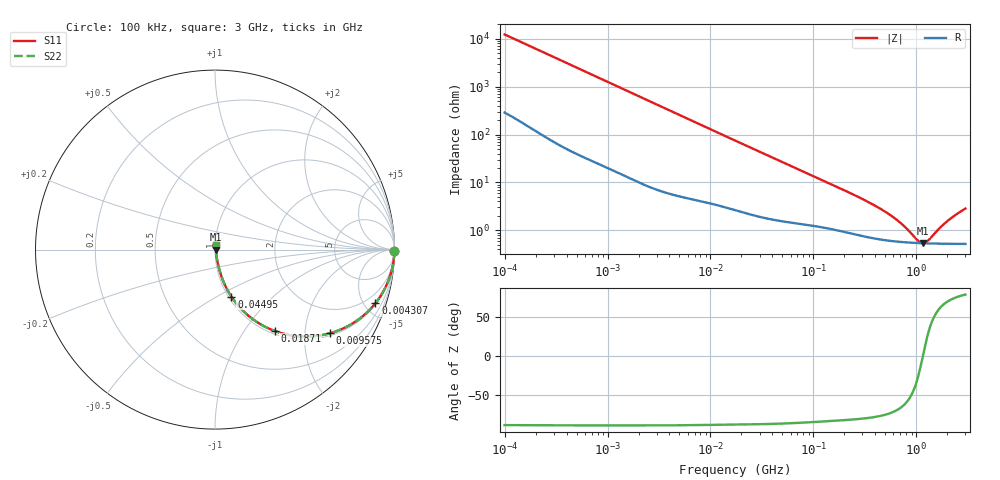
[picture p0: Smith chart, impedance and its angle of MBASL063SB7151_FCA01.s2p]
! MBASL063SB7151_FCA01  S-PARAMETER MODEL  ( Standard Model )
! Model Generated by TAIYO YUDEN Corporation (http://www.ty-top.com)
! Version 3.0
! TAIYO YUDEN Control No. 231201
! Copyright(c) 2020 TAIYO YUDEN CO.,LTD. All Rights Reserved.
! Product Description (link to TY-COMPAS)
! https://ds.yuden.co.jp/TYCOMPAS/or/detail?pn=MBASL063SB7151KFCA01&u=M
! Products Name : Multilayer Ceramic Capacitors
! Characteristics :
!  Capacitance : 150 [pF] , Rated Voltage : 10 [V] , TCC : X7R
!  Case Size : 0.6 x 0.3 / 0.024 x 0.012 [mm/inch] , Thickness : 0.3 / 0.012 [mm/inch]
!  (Conditions: Temperature = 25 [degC] , DC Bias Voltage = 0 [V])
! External Node Assignments :
!  1  o---| |---o  2
! GND o---------o GND
! Frequency Range : 100kHz  -  3GHz  [ 401 STEP ]
# MHZ S RI R 50
! Freq[MHz].  S11 Real  S11 Imag  S21 Real  S21 Imag  S12 Real  S12 Imag  S22 Real  S22 Imag
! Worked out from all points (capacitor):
!   401 points, 100 kHz to 3 GHz, reference 50 ohm
!   read as one part in series: C = 129 pF near 105.3 kHz
!   lowest |Z| = 537 mohm at 1.156 GHz (marker M1)
!   series resonance near 1.157 GHz, so ESL is about 150 pH
!   S11 on the Smith chart (normalised r, x): 100 kHz: open; 4.307 MHz: 1.11, -5.93; 9.575 MHz: 1.07, -2.69; 18.71 MHz: 1.05, -1.39; 44.95 MHz: 1.03, -0.59; 3 GHz: 1.01, +0.06
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0.1  0.9997 -0.00811  0.000256 0.00811  0.000256 0.00811  0.9997 -0.00811
0.562235  0.9973 -0.0446  0.0027 0.0446  0.0027 0.0446  0.9973 -0.0446
1.458987  0.9852 -0.1133  0.0148 0.1133  0.0148 0.1133  0.9852 -0.1133
3.161081  0.9385 -0.2319  0.0615 0.2319  0.0615 0.2319  0.9385 -0.2319
4.306746  0.8933 -0.2995  0.1067 0.2995  0.1067 0.2995  0.8933 -0.2995
6.3393  0.7978 -0.3905  0.2022 0.3905  0.2022 0.3905  0.7978 -0.3905
9.574722  0.6402 -0.4663  0.3598 0.4663  0.3598 0.4663  0.6402 -0.4663
13.04487  0.4962 -0.4844  0.5038 0.4844  0.5038 0.4844  0.4962 -0.4844
17.7727  0.354 -0.4608  0.646 0.4608  0.646 0.4608  0.354 -0.4608
18.71281  0.3321 -0.4532  0.6679 0.4532  0.6679 0.4532  0.3321 -0.4532
29.00125  0.1802 -0.3634  0.8198 0.3634  0.8198 0.3634  0.1802 -0.3634
44.94634  0.0915 -0.2623  0.9085 0.2623  0.9085 0.2623  0.0915 -0.2623
97.38194  0.0302 -0.1317  0.9698 0.1317  0.9698 0.1317  0.0302 -0.1317
294.964  0.00957 -0.0444  0.9904 0.0444  0.9904 0.0444  0.00957 -0.0444
547.5153  0.00643 -0.0203  0.9936 0.0203  0.9936 0.0203  0.00643 -0.0203
745.9503  0.00576 -0.0113  0.9942 0.0113  0.9942 0.0113  0.00576 -0.0113
1042.837  0.0054 -0.0026  0.9946 0.0026  0.9946 0.0026  0.0054 -0.0026
1156.079  0.00534 -1.49e-05  0.9947 1.49e-05  0.9947 1.49e-05  0.00534 -1.49e-05
1315.078  0.00531 0.00323  0.9947 -0.00323  0.9947 -0.00323  0.00531 0.00323
1701.687  0.00533 0.00994  0.9947 -0.00994  0.9947 -0.00994  0.00533 0.00994
2091.327  0.00545 0.0158  0.9946 -0.0158  0.9946 -0.0158  0.00545 0.0158
3000  0.00594 0.0277  0.9941 -0.0277  0.9941 -0.0277  0.00594 0.0277
